TYPE ST_STLHmiData :
STRUCT
	bInCommissioning				: BOOL;		// command signal commissioning mode (on rising edge)
	bInCommissioningRedLightOn		: BOOL;		// test signal to toggle red light state (true/false -> on/off) 
	bInCommissioningYellowLightOn	: BOOL;		// test signal to toggle yellow light on (true/false -> on/off)
	bInCommissioningGreenLightOn	: BOOL;		// test signal to toggle green light on (true/false -> on/off)
	bInAutomatic					: BOOL;		// command signal automatic mode (on rising edge)
	bInAutomaticActive				: BOOL;		// command signal automatic active mode (on rising edge) -> red and green on request
	bInAutoActiveRedRequest			: BOOL;		// command signal request red (on rising edge)
	bInAutoActiveGreenRequest		: BOOL;		// command signal request green (on rising edge)
	bInAutomaticStandBy				: BOOL;		// command signal automatic stand by mode (on rising edge) -> yellow light blinks 
	bOutCommissioningMode			: BOOL;		// status signal commissioning mode active
	bOutAutomaticMode				: BOOL;		// status signal automatic mode active
	bOutAutomaticActiveMode			: BOOL;		// status signal automatic active mode active
	sOutName						: STRING;	// name of traffic light
	bOutRedLightStatus				: BOOL;		// status signal red light
	bOutYellowLightStatus			: BOOL;		// status signal yellow light
	bOutGreenLightStatus			: BOOL;		// status signal green light
END_STRUCT
END_TYPE
